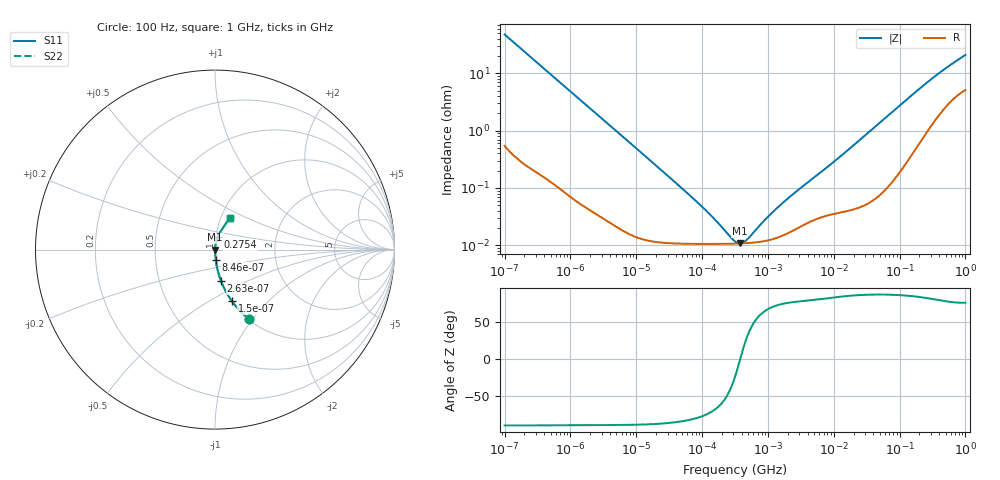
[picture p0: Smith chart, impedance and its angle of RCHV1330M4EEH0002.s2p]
! RCHV1330M4EEH0002  S-PARAMETER MODEL  (AEC-Q200 qualified)
! Model Generated by ELNA Corporation (http://www.ty-top.com)
! Version 1.0
! ELNA Control No. 240229
! Copyright (c) 2024 ELNA CO.,LTD. All Rights Reserved.
! Products Name : CONDUCTIVE POLYMER HYBRID ALUMINUM ELECTROLYTIC CAPACITORS
! Characteristics :
!  Capacitance  :  33uF  ,  Rated voltage  :  63V
!  Operating Temp. Range  :  -55 to +105 degC  ,  Endurance  :  5000hr at 105 degC
!  Dimension D  :  8mm  ,  Dimension L  :  10mm
! Frequency Range : 100Hz - 1GHz
! External Node Assignments :
!  1  o---| |---o  2
# MHz S RI R 50
!Freq[MHz].  S11 Real  S11 Imag  S21 Real  S21 Imag  S12 Real  S12 Imag  S22 Real  S22 Imag
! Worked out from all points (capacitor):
!   401 points, 100 Hz to 1 GHz, reference 50 ohm
!   read as one part in series: C = 33.4 uF near 108 Hz
!   lowest |Z| = 10.8 mohm at 371.5 kHz (marker M1)
!   series resonance near 379.4 kHz, so ESL is about 5.3 nH
!   S11 on the Smith chart (normalised r, x): 100 Hz: 1.01, -0.95; 150 Hz: 1.01, -0.64; 263 Hz: 1.00, -0.36; 846 Hz: 1.00, -0.11; 275.4 MHz: 1.02, +0.14; 1 GHz: 1.10, +0.41
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0.0001  0.1874 -0.3846  0.8126 0.3846  0.8126 0.3846  0.1874 -0.3846
0.00015  0.0945 -0.2872  0.9055 0.2872  0.9055 0.2872  0.0945 -0.2872
0.000263  0.0338 -0.175  0.9662 0.175  0.9662 0.175  0.0338 -0.175
0.000462  0.0119 -0.1023  0.9881 0.1023  0.9881 0.1023  0.0119 -0.1023
0.000846  0.00403 -0.0567  0.996 0.0567  0.996 0.0567  0.00403 -0.0567
0.001488  0.00156 -0.0325  0.9984 0.0325  0.9984 0.0325  0.00156 -0.0325
0.022131  0.000117 -0.00222  0.9999 0.00222  0.9999 0.00222  0.000117 -0.00222
0.106537  0.000106 -0.000426  0.9999 0.000426  0.9999 0.000426  0.000106 -0.000426
0.153109  0.000106 -0.000269  0.9999 0.000269  0.9999 0.000269  0.000106 -0.000269
0.316228  0.000107 -4.74e-05  0.9999 4.74e-05  0.9999 4.74e-05  0.000107 -4.74e-05
0.371535  0.000107 -5.35e-06  0.9999 5.35e-06  0.9999 5.35e-06  0.000107 -5.35e-06
0.419276  0.000108 2.6e-05  0.9999 -2.6e-05  0.9999 -2.6e-05  0.000108 2.6e-05
0.473151  0.000109 5.77e-05  0.9999 -5.77e-05  0.9999 -5.77e-05  0.000109 5.77e-05
0.865964  0.000118 0.000237  0.9999 -0.000237  0.9999 -0.000237  0.000118 0.000237
1.348963  0.000134 0.000416  0.9999 -0.000416  0.9999 -0.000416  0.000134 0.000416
2.371374  0.000179 0.000748  0.9998 -0.000748  0.9998 -0.000748  0.000179 0.000748
4.704354  0.000269 0.00141  0.9997 -0.00141  0.9997 -0.00141  0.000269 0.00141
13.4122  0.000392 0.00375  0.9996 -0.00375  0.9996 -0.00375  0.000392 0.00375
69.9842  0.00147 0.0191  0.9985 -0.0191  0.9985 -0.0191  0.00147 0.0191
275.4229  0.0152 0.0699  0.9848 -0.0699  0.9848 -0.0699  0.0152 0.0699
524.8075  0.0406 0.1159  0.9594 -0.1159  0.9594 -0.1159  0.0406 0.1159
1000  0.0828 0.1772  0.9172 -0.1772  0.9172 -0.1772  0.0828 0.1772
